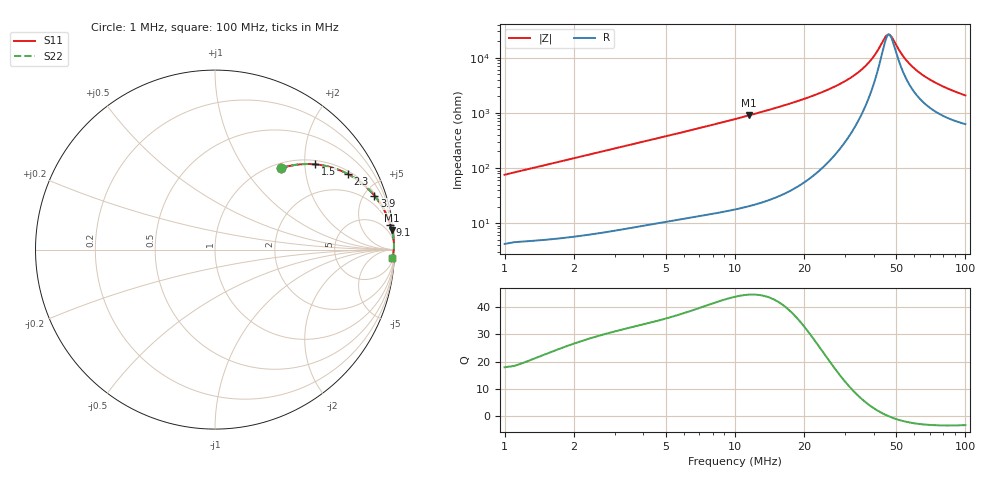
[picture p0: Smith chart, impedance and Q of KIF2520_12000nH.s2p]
!version-2
!date-12.2020
!Series
# MHz S RI R 50
!Freq ReS11 ImS11 ReS21 ImS21 ReS12 ImS12 ReS22 ImS22
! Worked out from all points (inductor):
!   991 points, 1 MHz to 100 MHz, reference 50 ohm
!   read as one part in series: L = 11.9 uH near 1.4 MHz
!   highest Q = 44.3 at 11.5 MHz (marker M1), where L = 12.5 uH
!   self-resonance near 46.69 MHz
!   S11 on the Smith chart (normalised r, x): 1 MHz: 1.08, +1.50; 1.5 MHz: 1.10, +2.26; 2.3 MHz: 1.12, +3.46; 3.9 MHz: 1.18, +5.85; 9.1 MHz: 1, +14; 100 MHz: 13, -40
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1  0.3689 0.4554  0.6311 -0.4554  0.6311 -0.4554  0.3689 0.4554
1.5  0.5584 0.475  0.4416 -0.475  0.4416 -0.475  0.5584 0.475
2.3  0.7421 0.4201  0.2579 -0.4201  0.2579 -0.4201  0.7421 0.4201
3  0.8276 0.3619  0.1724 -0.3619  0.1724 -0.3619  0.8276 0.3619
3.9  0.8884 0.3002  0.1116 -0.3002  0.1116 -0.3002  0.8884 0.3002
6.2  0.9513 0.2024  0.0487 -0.2024  0.0487 -0.2024  0.9513 0.2024
9.1  0.9767 0.1396  0.0233 -0.1396  0.0233 -0.1396  0.9767 0.1396
11.5  0.9854 0.1092  0.0146 -0.1092  0.0146 -0.1092  0.9854 0.1092
17.5  0.9938 0.0663  0.00618 -0.0663  0.00618 -0.0663  0.9938 0.0663
28.5  0.9971 0.0298  0.00287 -0.0298  0.00287 -0.0298  0.9971 0.0298
34  0.9973 0.0186  0.00274 -0.0186  0.00274 -0.0186  0.9973 0.0186
39.3  0.997 0.00998  0.00301 -0.00998  0.00301 -0.00998  0.997 0.00998
44.5  0.9965 0.00276  0.00352 -0.00276  0.00352 -0.00276  0.9965 0.00276
45.7  0.9963 0.00123  0.00366 -0.00123  0.00366 -0.00123  0.9963 0.00123
47.4  0.9961 -0.000862  0.00388 0.000862  0.00388 0.000862  0.9961 -0.000862
50.5  0.9957 -0.00448  0.00433 0.00448  0.00433 0.00448  0.9957 -0.00448
53.6  0.9952 -0.00788  0.00483 0.00788  0.00483 0.00788  0.9952 -0.00788
57.2  0.9945 -0.0116  0.00546 0.0116  0.00546 0.0116  0.9945 -0.0116
61.6  0.9937 -0.0158  0.00631 0.0158  0.00631 0.0158  0.9937 -0.0158
67  0.9925 -0.0207  0.00745 0.0207  0.00745 0.0207  0.9925 -0.0207
83.5  0.9885 -0.0336  0.0115 0.0336  0.0115 0.0336  0.9885 -0.0336
100  0.9837 -0.0446  0.0163 0.0446  0.0163 0.0446  0.9837 -0.0446
